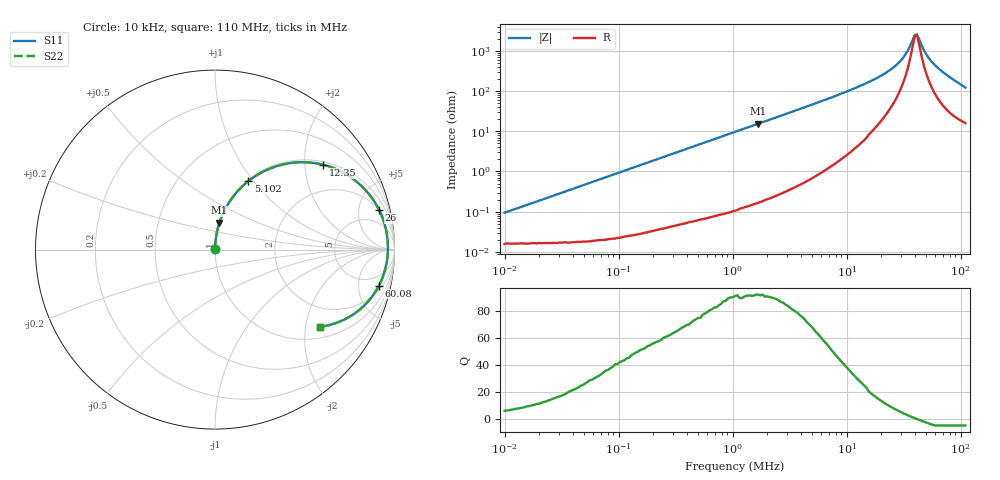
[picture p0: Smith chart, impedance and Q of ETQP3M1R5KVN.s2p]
! *** S-Parameter ***
!Copyright (C)  Panasonic Industry Corporation
!Power Inductors for Automotive application
!Parts No. ETQP3M1R5KVN
# HZ S RI R 50.000000
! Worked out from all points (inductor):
!   201 points, 10 kHz to 110 MHz, reference 50 ohm
!   read as one part in series: L = 1.49 uH near 10.48 kHz
!   highest Q = 92.2 at 1.67 MHz (marker M1), where L = 1.46 uH
!   self-resonance near 39.52 MHz
!   S11 on the Smith chart (normalised r, x): 10 kHz: 1.00, +0.00; 5.102 MHz: 1.01, +0.95; 12.35 MHz: 1.08, +2.48; 26 MHz: 2.04, +7.86; 60.08 MHz: 2.63, -8.42; 110 MHz: 1.32, -2.41
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10000  0.000159 0.000936  0.9998 -0.000936  0.9998 -0.000936  0.000159 0.000936
48644.84  0.000202 0.00453  0.9998 -0.00453  0.9998 -0.00453  0.000202 0.00453
225874.2  0.000799 0.0209  0.9992 -0.0209  0.9992 -0.0209  0.000799 0.0209
1048809  0.0102 0.0952  0.9898 -0.0952  0.9898 -0.0952  0.0102 0.0952
1670190  0.0245 0.1492  0.9755 -0.1492  0.9755 -0.1492  0.0245 0.1492
3203786  0.0825 0.2692  0.9175 -0.2692  0.9175 -0.2692  0.0825 0.2692
5101914  0.1864 0.382  0.8136 -0.382  0.8136 -0.382  0.1864 0.382
8511570  0.3995 0.4788  0.6005 -0.4788  0.6005 -0.4788  0.3995 0.4788
1.234996e7  0.6035 0.4727  0.3965 -0.4727  0.3965 -0.4727  0.6035 0.4727
1.79193e7  0.7897 0.3779  0.2103 -0.3779  0.2103 -0.3779  0.7897 0.3779
2.368988e7  0.8902 0.2642  0.1098 -0.2642  0.1098 -0.2642  0.8902 0.2642
2.600021e7  0.9143 0.2213  0.0857 -0.2213  0.0857 -0.2213  0.9143 0.2213
2.989494e7  0.9413 0.1543  0.0587 -0.1543  0.0587 -0.1543  0.9413 0.1543
3.281041e7  0.9535 0.1084  0.0465 -0.1084  0.0465 -0.1084  0.9535 0.1084
3.60102e7  0.9609 0.0618  0.0391 -0.0618  0.0391 -0.0618  0.9609 0.0618
3.952205e7  0.9637 0.0147  0.0363 -0.0147  0.0363 -0.0147  0.9637 0.0147
4.14044e7  0.9633 -0.00902  0.0367 0.00902  0.0367 0.00902  0.9633 -0.00902
4.544231e7  0.959 -0.0567  0.041 0.0567  0.041 0.0567  0.959 -0.0567
4.987401e7  0.9495 -0.1046  0.0505 0.1046  0.0505 0.1046  0.9495 -0.1046
6.007616e7  0.9136 -0.2002  0.0864 0.2002  0.0864 0.2002  0.9136 -0.2002
7.942257e7  0.8067 -0.3341  0.1933 0.3341  0.1933 0.3341  0.8067 -0.3341
1.1e8  0.5854 -0.431  0.4146 0.431  0.4146 0.431  0.5854 -0.431
